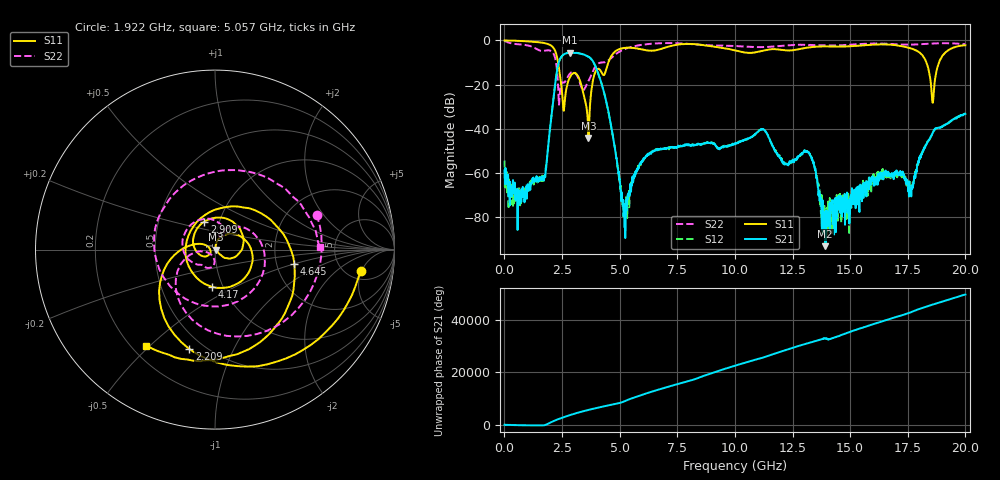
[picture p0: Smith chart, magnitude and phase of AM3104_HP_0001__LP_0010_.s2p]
!Created with skrf (http://scikit-rf.org).
# Hz S RI R 50.0
!freq ReS11 ImS11 ReS21 ImS21 ReS12 ImS12 ReS22 ImS22
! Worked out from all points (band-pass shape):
!   1601 points, 10 MHz to 20 GHz, reference 50 ohm
!   highest |S21| = -5.53 dB at 2.846 GHz (marker M1); lowest = -93.2 dB at 13.92 GHz (marker M2)
!   |S21| within 3 dB of the highest: 2.409 GHz to 3.777 GHz (1.367 GHz wide, 44.2 % of centre)
!   lowest |S11| = -44.2 dB at 3.646 GHz (marker M3), VSWR 1.01, Z = 50.6 + j0.00491 ohm
!   |S11| at or under -10 dB: 2.328 GHz to 4.511 GHz (2.182 GHz wide, 63.8 % of centre); 18.31 GHz to 18.85 GHz (546.7 MHz wide, 2.94 % of centre)
!   |S22| runs from -29.1 to -0.2 dB; largest |S21 - S12| = 0.0043
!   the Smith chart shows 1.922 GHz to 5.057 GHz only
!   S11 on the Smith chart (normalised r, x): 1.922 GHz: 6.59, -4.80; 2.209 GHz: 0.42, -0.69; 2.909 GHz: 0.85, +0.27; 4.17 GHz: 0.89, -0.39; 4.645 GHz: 2.51, -0.50; 5.057 GHz: 0.26, -0.49
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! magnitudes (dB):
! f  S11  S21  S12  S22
! 10 MHz  0.0  -58.8  -54.4  -0.2
! 759.6 MHz  -0.2  -70.9  -69.2  -1.8
! 1.697 GHz  -1.1  -61.7  -62.2  -4.7
! 1.922 GHz  -1.7  -45.4  -45.7  -4.5
! 2.209 GHz  -4.9  -19.2  -19.2  -8.3
! 2.559 GHz  -31.1  -6.5  -6.5  -19.0
! 2.846 GHz  -16.6  -5.5  -5.6  -15.0
! 2.909 GHz  -15.5  -5.6  -5.6  -14.4
! 3.346 GHz  -20.6  -6.1  -6.1  -21.4
! 3.646 GHz  -44.2  -7.4  -7.4  -18.4
! 4.17 GHz  -13.6  -18.0  -18.0  -10.0
! 4.645 GHz  -7.0  -39.6  -39.7  -7.9
! 5.057 GHz  -3.6  -68.0  -67.2  -4.7
! 5.232 GHz  -3.3  -74.3  -80.2  -3.8
! 6.682 GHz  -4.2  -49.6  -49.4  -1.3
! 10.01 GHz  -4.4  -46.6  -46.7  -2.5
! 13.34 GHz  -2.9  -53.1  -54.0  -2.1
! 13.92 GHz  -2.7  -93.2  -87.5  -2.2
! 16.68 GHz  -1.8  -60.9  -61.9  -1.5
! 17.63 GHz  -3.6  -69.2  -68.3  -1.9
! 18.58 GHz  -28.2  -42.2  -41.9  -1.4
! 20 GHz  -2.2  -33.3  -33.2  -1.7
